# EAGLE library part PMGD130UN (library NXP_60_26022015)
20 V, dual N-channel Trench MOSFET AAL Eindhoven MK
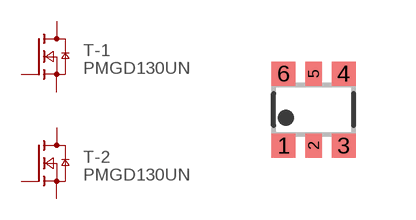
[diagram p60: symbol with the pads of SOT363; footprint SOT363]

Designator prefix T; gates -1=N-MOSFET -2=N-MOSFET

## PMGD130UN  [SOT363]
1  -1:S  pas
2  -1:G  pas
3  -2:D  pas
4  -2:S  pas
5  -2:G  pas
6  -1:D  pas

## Footprint SOT363 (pad centres in mm)
SOT363 Plastic surface-mounted package; 6 leads JEDEC: -- IEC: -- JEITA: SC-88
smd 0.6 x 0.6: 1 -0.75,-0.9; 3 0.75,-0.9; 4 0.75,0.9; 6 -0.75,0.9
smd 0.4 x 0.6: 2 0,-0.9; 5 0,0.9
